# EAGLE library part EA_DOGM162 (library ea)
ELECTRONIC ASSEMBYL GmbH EA DOGM162-A EA DOGM081-A EA DOGM163-A
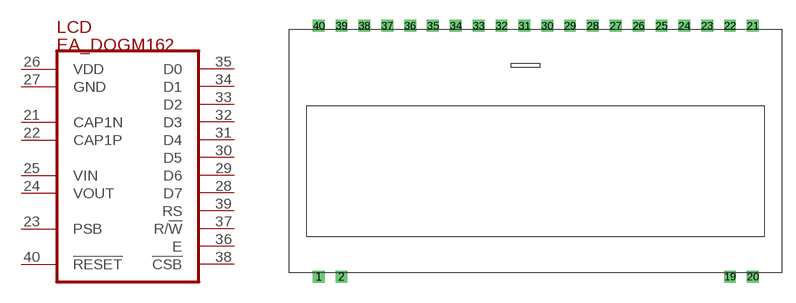
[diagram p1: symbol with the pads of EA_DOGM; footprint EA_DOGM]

Designator prefix LCD

## EA_DOGM162  [EA_DOGM]
21  CAP1N  pas
22  CAP1P  pas
23  PSB  in
24  VOUT  pas
25  VIN  pas
26  VDD  pwr
27  GND  pwr
28  D7
29  D6
30  D5
31  D4
32  D3
33  D2
34  D1
35  D0
36  E  in
37  R/!W!  in
38  !CSB!  in
39  RS  in
40  !RESET!  in

## Footprint EA_DOGM (pad centres in mm)
EA DOM081 / EA DOGM162 / EA DOGM163 Textdisplays COG inkl.Kontroller Hersteller: ELECTRONIC ASSEMBLY GmbH http://www.lcd-module.de
drill 0.813 square: 1 0,0; 2 2.54,0; 19 45.72,0; 20 48.26,0; 21 48.26,27.94; 22 45.72,27.94; 23 43.18,27.94; 24 40.64,27.94; 25 38.1,27.94; 26 35.56,27.94; 27 33.02,27.94; 28 30.48,27.94; 29 27.94,27.94; 30 25.4,27.94; 31 22.86,27.94; 32 20.32,27.94; 33 17.78,27.94; 34 15.24,27.94; 35 12.7,27.94; 36 10.16,27.94; 37 7.62,27.94; 38 5.08,27.94; 39 2.54,27.94; 40 0,27.94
